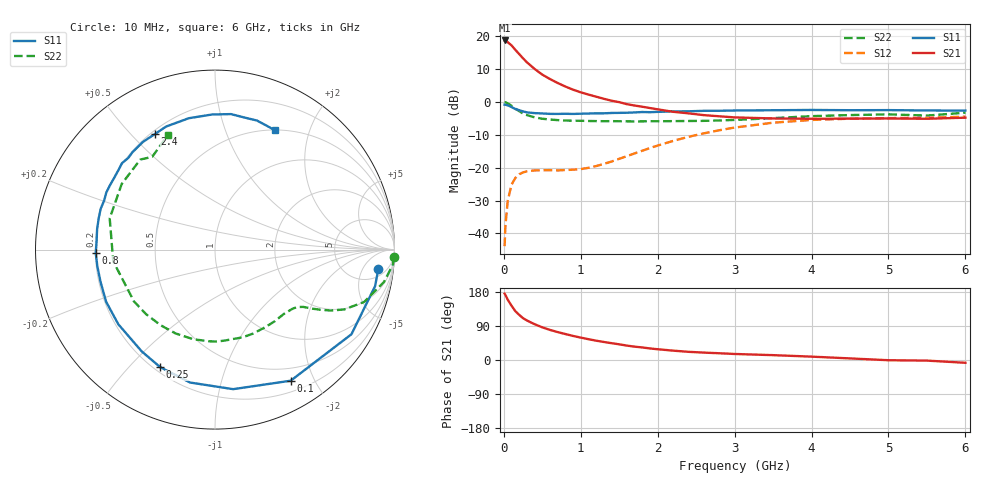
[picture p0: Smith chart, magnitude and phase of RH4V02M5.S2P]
! SIEMENS Small Signal Semiconductors
! BFR106
! Si NPN RF Bipolar Junction Transistor in SOT23
! VCE = 4 V  IC = 2.5 mA
! Common Emitter S-Parameters:  August  1996
# GHz  S  MA  R  50
!  f  S11  S21  S12  S22
! GHz  MAG  ANG  MAG  ANG  MAG  ANG  MAG  ANG
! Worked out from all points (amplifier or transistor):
!   36 points, 10 MHz to 6 GHz, reference 50 ohm
!   highest |S21| = 18.8 dB at 10 MHz (marker M1)
!   |S21| within 3 dB of that: start of sweep to 155 MHz
!   unconditionally stable (mu >= 1): 745.8 MHz to 1.933 GHz; 4.139 GHz to end of sweep
!   at 250 MHz: K = 0.35, MSG = 17.4 dB, |S12| = -21.4 dB
!   at 1.4 GHz: K = 1.23, MAG = 6.4 dB, |S12| = -18.1 dB
!   at 6 GHz: K = 1.02, MAG = -1.0 dB, |S12| = -4.4 dB
!   S11 on the Smith chart (normalised r, x): 10 MHz: 8, -11; 100 MHz: 0.33, -1.68; 250 MHz: 0.22, -0.61; 800 MHz: 0.20, -0.01; 2.4 GHz: 0.22, +0.59; 6 GHz: 0.50, +1.50
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0.01  0.9166 -6.6  8.703 175.1  0.0064 88.0  0.9961 -2.4
0.02  0.9148 -12.9  8.64 171.8  0.013 82.2  0.995 -4.7
0.05  0.8947 -31.8  8.198 159.4  0.0312 72.3  0.9593 -10.8
0.1  0.8435 -60.0  7.312 143.2  0.0554 59.4  0.8811 -19.3
0.15  0.7841 -82.6  6.253 128.7  0.0701 48.1  0.7946 -24.8
0.2  0.7535 -100.6  5.392 119.0  0.0797 41.4  0.7284 -27.8
0.25  0.7226 -115.0  4.648 110.4  0.0852 36.6  0.6708 -29.9
0.3  0.6989 -125.7  4.044 104.3  0.0883 33.6  0.6354 -31.2
0.4  0.6806 -142.3  3.202 94.4  0.0913 29.7  0.5861 -33.0
0.5  0.6726 -154.4  2.624 86.2  0.0919 28.7  0.5588 -34.9
0.6  0.6626 -164.2  2.248 79.4  0.0921 29.7  0.543 -37.4
0.8  0.6648 -178.3  1.728 68.5  0.0924 35.0  0.5247 -43.3
1.1  0.6709 165.0  1.304 54.9  0.1 48.4  0.5164 -53.9
1.6  0.6897 144.3  0.931 38.0  0.1505 65.3  0.5105 -74.7
2.2  0.7219 123.8  0.713 24.7  0.2566 65.4  0.5139 -103.8
2.4  0.7257 117.5  0.675 21.6  0.2963 62.5  0.5162 -115.1
3.5  0.7529 91.2  0.564 12.8  0.4867 38.8  0.5707 -173.4
4  0.7602 83.3  0.558 8.9  0.5356 27.3  0.6118 163.5
4.5  0.7537 76.9  0.561 4.2  0.5596 17.3  0.6354 144.9
5  0.7562 72.0  0.564 -0.6  0.5721 9.0  0.652 129.7
5.5  0.747 66.7  0.558 -1.6  0.5769 5.0  0.6242 124.1
6  0.7437 63.4  0.58 -7.4  0.6014 -3.0  0.6905 112.3
